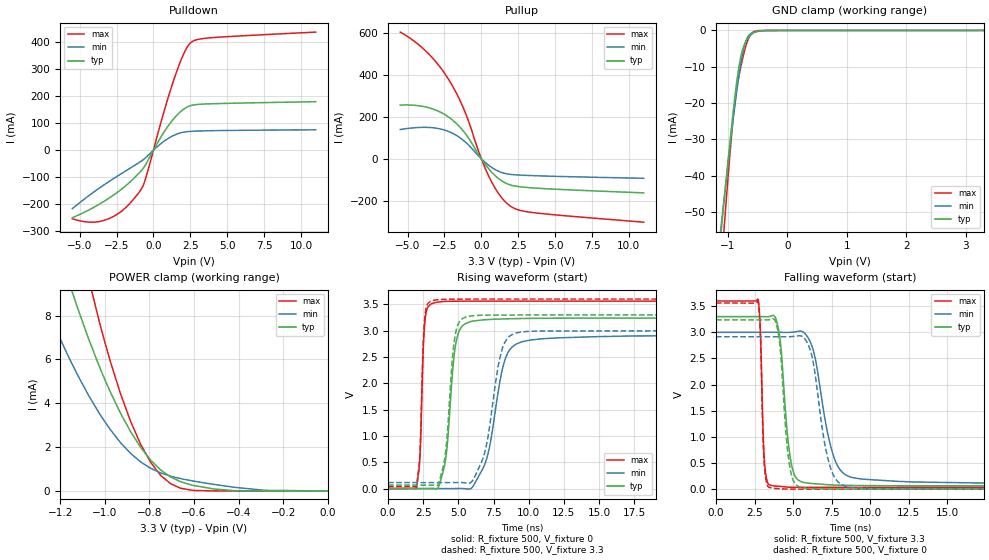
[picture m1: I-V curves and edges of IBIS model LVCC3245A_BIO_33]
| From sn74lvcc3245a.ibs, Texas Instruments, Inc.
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[Model]   LVCC3245A_BIO_33
Model_type  I/O
Vinl=0.8
Vinh=2.0
Enable   Active-Low
Vref =   0
Rref =   500
Cref =   50p
Vmeas =   1.5
| variable   typ   min   max
C_comp   18.50pF   NA   NA
| C_pullup   13.90pF   8.68pF   18.93pF
| C_pulldown   8.47pF   3.05pF   13.09pF
| C_tri-state   7.79pF   6.74pF   8.78pF
[Temperature Range]   40   100   -40
| Ambient temperature   25   85   -40
[Voltage range]   3.3   3   3.6
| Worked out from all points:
|   slope of the pulldown table from 0 to 0.495 V, typ, clamps not added: 10.4 ohm
|   slope of the pullup table from 0 to 0.495 V, typ, clamps not added: 10.5 ohm
|   GND clamp passes 1 mA (typ) near -0.60 V on its own axis
|   POWER clamp passes 1 mA (typ) near -0.75 V on its own axis
|   rising waveform, R_fixture 500, V_fixture 0: 20-80 % time 587ps typ, 1.16ns min, 252ps max; typ from 0 V to 3.24 V
|   falling waveform, R_fixture 500, V_fixture 3.3: 20-80 % time 535ps typ, 1.07ns min, 205ps max; typ from 3.3 V to 0.064 V
|   rising waveform, R_fixture 500, V_fixture 3.3: 20-80 % time 544ps typ, 1.03ns min, 242ps max; typ from 0.064 V to 3.3 V
|   falling waveform, R_fixture 500, V_fixture 0: 20-80 % time 487ps typ, 901ps min, 196ps max; typ from 3.24 V to 0 V
[GND Clamp]
| LVCC3245A_BIO_33
|   Voltage   I(typ)   I(min)   I(max)
-5.5V     -941.9mA   -838.1mA   -1.112A
-1.145V   -60.94mA   -58.72mA   -72.38mA
-1.1V     -53.17mA   -51.88mA   -62.42mA
-1.06V    -46.36mA   -45.87mA   -53.7mA
-930mV    -25.27mA   -27.08mA   -27.39mA
-855mV    -14.67mA   -17.18mA   -16.58mA
-785mV    -7.394mA   -9.264mA   -10.21mA
-725mV    -4.03mA    -4.345mA   -5.867mA
-665mV    -2.21mA    -1.749mA   -2.681mA
-585mV    -848.2uA   -614.5uA   -572.4uA
-330mV    -6.802uA   -44.23uA   -535.4nA
3.3V      1.644nA    37.51uA    26.59pA
[POWER Clamp]
| LVCC3245A_BIO_33
|   Voltage   I(typ)   I(min)   I(max)
-5.5V     376.1mA    259.6mA    632.7mA
-1.285V   13.82mA    8.979mA    20.69mA
-1.155V   9.363mA    5.967mA    13.54mA
-1.125V   8.444mA    5.355mA    12.07mA
-1.075V   7.01mA     4.405mA    9.803mA
-1.025V   5.697mA    3.55mA     7.745mA
-975mV    4.512mA    2.796mA    5.908mA
-840mV    2.001mA    1.33mA     2.143mA
-795mV    1.414mA    1.035mA    1.314mA
-705mV    634.9uA    672.5uA    329.3uA
-510mV    88.78uA    296.1uA    1.009uA
-95.1fV   1.644nA    10.03nA    31.19pA
[Pulldown]
| LVCC3245A_BIO_33
|   Voltage   I(typ)   I(min)   I(max)
-5.5V     -249.1mA   -215.9mA   -253.5mA
-4.18V    -215.1mA   -159.8mA   -266mA
-3.02V    -177.4mA   -116.1mA   -252.7mA
-1.92V    -133.3mA   -78.1mA    -214.1mA
-880mV    -79.11mA   -42.57mA   -148mA
-535mV    -53.63mA   -27.86mA   -104.9mA
695mV     64.86mA    31.99mA    138.8mA
1.46V     121.3mA    56.52mA    272.6mA
2.095V    153mA      66.87mA    360.7mA
2.575V    165mA      69.5mA     398.7mA
3.91V     171.1mA    71.77mA    414.9mA
11V       178.9mA    75.1mA     435.8mA
[Pullup]
| LVCC3245A_BIO_33
|   Voltage   I(typ)   I(min)   I(max)
-5.5V     256.2mA    139.9mA    603.8mA
-3.705V   246mA      150.1mA    509.2mA
-2.93V    227.6mA    144.6mA    448.9mA
-2.23V    199.5mA    130.5mA    379.3mA
-1.17V    127.5mA    85.26mA    233.5mA
-75mV     8.09mA     5.357mA    13.91mA
515mV     -48.85mA   -31.7mA    -84.53mA
1.185V    -94.97mA   -59.65mA   -167.1mA
1.865V    -122mA     -73.08mA   -219.9mA
2.47V     -131.6mA   -76.7mA    -242.2mA
3.48V     -138.3mA   -79.89mA   -255.6mA
11V       -162mA     -92.6mA    -301.6mA
[Ramp]
| LVCC3245A_BIO_33
| variable   typ   min   max
dV/dt_r   1.95/5.91E-10   1.76/1.17E-09   2.14/2.56E-10
dV/dt_f   1.96/5.41E-10   1.75/1.08E-09   2.16/2.12E-10
R_load = 500
[Rising Waveform]
| LVCC3245A_BIO_33
R_fixture =   500
C_fixture =   0
L_fixture =   0
V_fixture =   0
V_fixture_min = 0
V_fixture_max = 0
|   Time   V(typ)   V(min)   V(max)
0s        202.6pV    118.9nV    82.71pV
2.02ns    8.153uV    453.1nV    8.657mV
2.27ns    -8uV       43.51nV    626.5mV
2.6ns     -35.76uV   1.496uV    3.119V
3.085ns   1.39mV     -1.835uV   3.51V
4.02ns    440.3mV    -39.35uV   3.554V
4.77ns    2.678V     715.3uV    3.559V
5.51ns    3.134V     -4.353mV   3.56V
9.095ns   3.228V     2.743V     3.561V
24.99ns   3.238V     2.913V     3.561V
[Falling Waveform]
| LVCC3245A_BIO_33
R_fixture =   500
C_fixture =   0
L_fixture =   0
V_fixture =   3.3
V_fixture_min = 3
V_fixture_max = 3.6
|   Time   V(typ)   V(min)   V(max)
0s        3.3V       3V         3.6V
2.735ns   3.3V       3V         3.621V
2.89ns    3.3V       3V         2.938V
3.13ns    3.299V     3V         590.9mV
3.47ns    3.303V     3V         79.16mV
4.055ns   3.055V     2.999V     54.51mV
4.775ns   686.5mV    2.999V     37.48mV
5.445ns   153.4mV    3.023V     35.07mV
8.49ns    72.69mV    259.4mV    34.17mV
24.99ns   64.31mV    113.5mV    34.14mV
[Rising Waveform]
| LVCC3245A_BIO_33
R_fixture =   500
C_fixture =   0
L_fixture =   0
V_fixture =   3.3
V_fixture_min = 3
V_fixture_max = 3.6
|   Time   V(typ)   V(min)   V(max)
0s        64.3mV     113.2mV    34.14mV
2.02ns    64.31mV    113.2mV    42.66mV
2.265ns   64.3mV     113.2mV    663.4mV
2.58ns    64.27mV    113.2mV    3.158V
3.01ns    65.02mV    113.2mV    3.555V
3.965ns   471.8mV    113.2mV    3.595V
4.695ns   2.775V     113.7mV    3.599V
5.32ns    3.232V     113.5mV    3.6V
8.805ns   3.297V     2.923V     3.6V
24.99ns   3.3V       2.999V     3.6V
[Falling Waveform]
| LVCC3245A_BIO_33
R_fixture =   500
C_fixture =   0
L_fixture =   0
V_fixture =   0
V_fixture_min = 0
V_fixture_max = 0
|   Time   V(typ)   V(min)   V(max)
0s        3.238V     2.915V     3.561V
2.73ns    3.238V     2.915V     3.584V
2.88ns    3.238V     2.915V     2.931V
3.115ns   3.237V     2.915V     541.8mV
3.44ns    3.24V      2.915V     34.86mV
4.03ns    2.998V     2.915V     8.992mV
4.695ns   613.3mV    2.914V     2.111mV
5.31ns    56.82mV    2.931V     1.045mV
8.185ns   2.01mV     79.39mV    67.91uV
24.99ns   1.155uV    49.73uV    258.5nV
